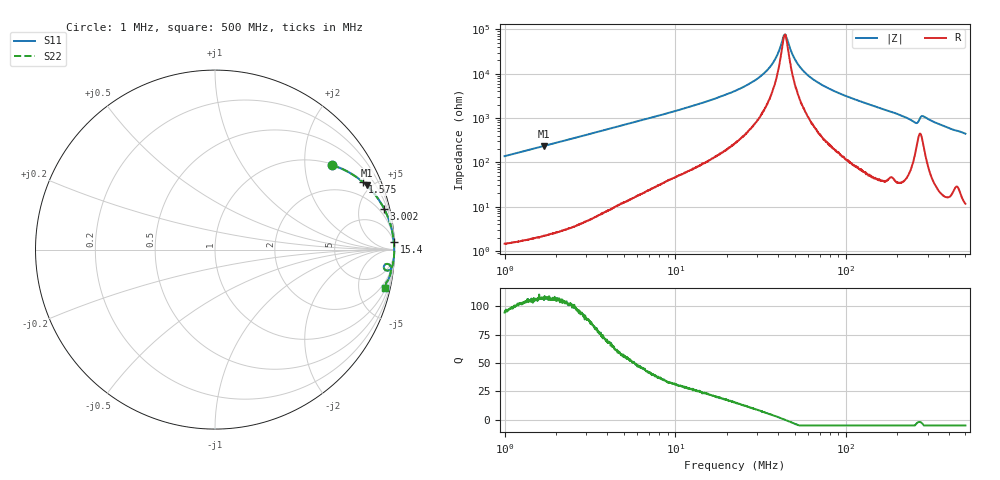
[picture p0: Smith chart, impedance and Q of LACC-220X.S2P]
!s-Parameter Generated by FASTRON Sdn. Bhd.
!FASTRON P/N : LACC-220X
!Keysight Technologies,E4991B,MY54100416,A.01.15
!Date: Wed Mar 18 09:36:09 2026
!Version  : Rev00 Wed Mar 18 09:36:09 2026
!Data & Calibration Information:
!PortZ  Port1:50+j0  Port2:50+j0
!When reading, reference impedance value at option line is always used.
!Remarks : This data is being provided solely for informational purposes.
!Freq	S11	S21	S12	S22
# Hz S dB R 50
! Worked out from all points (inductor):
!   1601 points, 1 MHz to 500 MHz, reference 50 ohm
!   read as one part in series: L = 21.9 uH near 1.032 MHz
!   highest Q = 108 at 1.709 MHz (marker M1), where L = 21.9 uH
!   self-resonance near 43.78 MHz
!   S11 on the Smith chart (normalised r, x): 1 MHz: 1.03, +2.75; 1.575 MHz: 1.04, +4.33; 3.002 MHz: 1.09, +8.29; 15.4 MHz: 3, +48; 500 MHz: 1.23, -8.83
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1000000  -1.89 35.8  -4.65 -53.6  -4.65 -53.6  -1.89 35.8
1575296  -0.87 24.7  -7.59 -64.8  -7.59 -64.8  -0.87 24.7
1709174  -0.75 23.0  -8.18 -66.5  -8.18 -66.5  -0.75 23.0
2820919  -0.30 14.4  -12.11 -75.0  -12.11 -75.0  -0.30 14.4
3001790  -0.27 13.5  -12.62 -75.8  -12.62 -75.8  -0.27 13.5
7957584  -0.05 5.1  -21.08 -83.4  -21.08 -83.4  -0.05 5.1
1.540092e7  -0.02 2.4  -27.59 -85.1  -27.59 -85.1  -0.02 2.4
2.236068e7  -0.02 1.4  -32.24 -84.8  -32.24 -84.8  -0.02 1.4
2.90071e7  -0.01 0.8  -36.80 -83.2  -36.80 -83.2  -0.01 0.8
3.481662e7  -0.01 0.5  -41.89 -79.2  -41.89 -79.2  -0.01 0.5
3.866622e7  -0.01 0.2  -46.95 -72.3  -46.95 -72.3  -0.01 0.2
4.260918e7  -0.01 0.1  -55.63 -36.0  -55.63 -36.0  -0.01 0.1
4.378357e7  -0.01 0.0  -57.63 -1.9  -57.63 -1.9  -0.01 0.0
4.499032e7  -0.01 -0.0  -56.07 33.1  -56.07 33.1  -0.01 -0.0
4.843613e7  -0.01 -0.2  -48.89 68.7  -48.89 68.7  -0.01 -0.2
5.154174e7  -0.01 -0.3  -44.96 76.3  -44.96 76.3  -0.01 -0.3
6.307767e7  -0.01 -0.7  -37.86 83.7  -37.86 83.7  -0.01 -0.7
9.08741e7  -0.01 -1.6  -31.22 85.8  -31.22 85.8  -0.01 -1.6
1.77937e8  -0.04 -4.0  -23.13 84.3  -23.13 84.3  -0.04 -4.0
2.543648e8  -0.29 -7.0  -18.15 71.1  -18.15 71.1  -0.29 -7.0
2.835887e8  -0.21 -5.0  -20.98 72.0  -20.98 72.0  -0.21 -5.0
5e8  -0.27 -12.7  -13.17 75.8  -13.17 75.8  -0.27 -12.7
